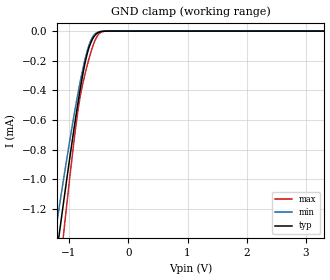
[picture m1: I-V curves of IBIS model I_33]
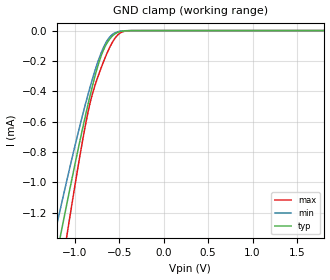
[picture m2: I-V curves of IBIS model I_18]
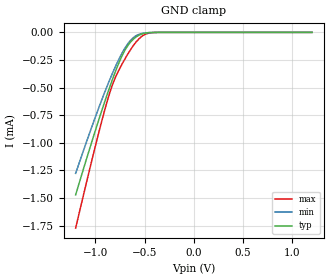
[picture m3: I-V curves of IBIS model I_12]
| TEXAS INSTRUMENTS INCORPORATED
| Standard Linear and Logic Group / High Volume Linear
| IBIS Model of TXB0304RSV, TXB0304RUT,
| 4 bit translator
| This file contains package information for the following:
|  RSV_16p 16-pin (PW) package as [Component] TXB0304RSV_PW
|  RUT_12 12-pin (PW) package as [Component] TXB0304RUT_PW
| This device can be powered at the following Vccs:
|  3.3 volt Vcc
|  1.8 volt Vcc
|  1.2 volt Vcc
| This file provides unique models under the [Model Selector] for each Vcc.
| For operation at a specific Vcc, select the appropriate model after each
| [Model Selector] keyword.
[IBIS Ver]   4.0
[Comment char]  |_char
[File Name]   txb0304.ibs
[File Rev]   1.1 | TXB0304
[Date]   June 21, 2012
[Source]   Data created from TI-SPICE simulations at TI-SLL/HVL.
   The following is an IBIS list for the TXB0304RSV and TXB0304RUT.
   Please contact sllibis@ti.com with questions and
   comments concerning SLL IBIS models.
[Notes]   Revision_History:
   - 1.1 06/21/12   Added models for one-shot circuit on for IO model
   - Non-monotonic behavior in I/O Pullup and Pulldown is expected
   -  Please note that models for one shot circuit on can be chosen under
   [Model Selector] for IO model.
[Disclaimer]
| This model is designed as an aid for customers of Texas Instruments.
| TI and its licensors and suppliers make no warranties, either expressed
| or implied, with respect to this  model, including the warranties of
| merchantability or fitness for a particular purpose. The model is
| provided solely on an "as is" basis. The entire risk as to its quality
| and performance is with the customer.
[Copyright]
| (C) Copyright 2012 Texas Instruments Incorporated. All rights reserved.
| Component TXB0304RSV_PW 16-PIN RSV_16P
[Component]   TXB0304RSV_PW
[Manufacturer]   Texas Instruments, Inc.
[Package]
|   typ   min   max
R_pkg   6.239e-02   1.070e-03   9.845e-02
L_pkg   6.891e-10   1.266e-10   1.063e-09
C_pkg   1.354e-13   8.974e-14   1.623e-13
[Pin]   signal_name   model_name   R_pin   L_pin   C_pin
1   A1   IO   7.350e-02   7.894e-10   1.363e-13
2   A2   IO   6.697e-02   7.142e-10   1.449e-13
3   A3   IO   6.675e-02   7.118e-10   1.438e-13
4   A4   IO   6.786e-02   7.288e-10   1.311e-13
5   NC   NC   1.070e-03   1.319e-10   8.974e-14
6   GND   GND   8.279e-02   8.839e-10   1.573e-13
7   GND   GND   8.757e-02   9.358e-10   1.623e-13
8   OE   I   9.845e-02   1.063e-09   1.529e-13
9   B4   IO   6.786e-02   7.222e-10   1.310e-13
10   B3   IO   6.675e-02   7.050e-10   1.436e-13
11   B2   IO   6.697e-02   7.075e-10   1.447e-13
12   B1   IO   7.350e-02   7.835e-10   1.361e-13
13   VCC   POWER   8.803e-02   9.463e-10   1.432e-13
14   NC   NC   1.070e-03   1.266e-10   1.031e-13
15   NC   NC   1.070e-03   1.266e-10   1.031e-13
16   VCC   POWER   8.803e-02   9.491e-10   1.433e-13
| Component TXB0304RUT_PW 12-PIN RUT_12
[Component]   TXB0304RUT_PW
[Manufacturer]   Texas Instruments, Inc.
[Package]
|   typ   min   max
R_pkg   6.179e-02   3.158e-02   6.816e-02
L_pkg   6.348e-10   4.117e-10   7.835e-10
C_pkg   2.231e-13   1.717e-13   2.693e-13
[Pin]   signal_name   model_name   R_pin   L_pin   C_pin
1   VCC   POWER   6.816e-02   7.779e-10   2.693e-13
2   A1   IO   6.153e-02   5.719e-10   1.863e-13
3   A2   IO   6.261e-02   5.772e-10   2.487e-13
4   A3   IO   6.455e-02   6.041e-10   1.874e-13
5   A4   IO   6.783e-02   7.745e-10   2.690e-13
6   GND   GND   3.158e-02   4.117e-10   1.880e-13
7   B4   IO   6.776e-02   7.764e-10   2.647e-13
8   B3   IO   6.455e-02   6.100e-10   1.875e-13
9   B2   IO   6.261e-02   5.835e-10   2.489e-13
10   B1   IO   6.153e-02   5.783e-10   1.865e-13
11   VCC   POWER   6.815e-02   7.835e-10   2.690e-13
12   OE   I   6.063e-02   5.684e-10   1.717e-13
| Model I
[Model Selector]   I
I_33   3.3 volt Vcc
I_18   1.8 volt Vcc
I_12   1.2 volt Vcc
| Model IO
[Model Selector]   IO
IO_33   3.3 volt Vcc
IO_18   1.8 volt Vcc
IO_12   1.2 volt Vcc
IO_33_OS   one shot circuit on at   3.3 volt Vcc
IO_18_OS   one shot circuit on at  1.8 volt Vcc
IO_12_OS   one shot circuit on at   1.2 volt Vcc
| Models and submodels in the file (9): I_33 (Input), I_18 (Input), I_12 (Input), IO_33 (3-state), IO_18 (3-state), IO_12 (3-state), IO_33_OS (I/O), IO_18_OS (I/O), IO_12_OS (I/O)
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[Model]   I_33
Model_type  Input
Vinl=1.155
Vinh=2.145
| variable   typ   min   max
C_comp   0.49pF   0.33pF   0.66pF
[Temperature Range]   40   100   -40
| Ambient temperature   25   85   -40
[Voltage range]   3.3   3   3.6
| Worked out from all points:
|   GND clamp passes 1 mA (typ) near -1.04 V on its own axis
[GND Clamp]
| I_33
|   Voltage   I(typ)   I(min)   I(max)
-3.3V     -8.236mA   -7.402mA   -10.23mA
-1.225V   -1.547mA   -1.344mA   -1.868mA
-1.16V    -1.353mA   -1.173mA   -1.622mA
-1.1V     -1.177mA   -1.018mA   -1.397mA
-1.075V   -1.104mA   -954.4uA   -1.305mA
-910mV    -642.5uA   -554.3uA   -721.3uA
-810mV    -387.9uA   -337.9uA   -438uA
-675mV    -126.6uA   -109.9uA   -203.7uA
-600mV    -51.19uA   -38.37uA   -103.3uA
-525mV    -14.23uA   -9.737uA   -34.33uA
-365mV    -261.1nA   -191.2nA   -391.1nA
3.3V      1.186nA    2.425nA    22.67pA
[Model]   I_18
Model_type  Input
Vinl=0.63
Vinh=1.17
| variable   typ   min   max
C_comp   0.53pF   0.36pF   0.72pF
[Temperature Range]   40   100   -40
| Ambient temperature   25   85   -40
[Voltage range]   1.8   1.65   1.95
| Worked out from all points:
|   GND clamp passes 1 mA (typ) near -1.04 V on its own axis
[GND Clamp]
| I_18
|   Voltage   I(typ)   I(min)   I(max)
-1.8V     -3.331mA   -2.937mA   -4.119mA
-1.22V    -1.532mA   -1.33mA    -1.85mA
-1.145V   -1.309mA   -1.134mA   -1.566mA
-1.075V   -1.104mA   -954.4uA   -1.305mA
-920mV    -669.4uA   -577.3uA   -754.3uA
-825mV    -424uA     -368.5uA   -472.8uA
-695mV    -155.3uA   -136.7uA   -234uA
-630mV    -76.03uA   -61.12uA   -140.6uA
-560mV    -27.36uA   -19.07uA   -61.57uA
-485mV    -6.022uA   -4.161uA   -14.74uA
-380mV    -401.2nA   -288.1nA   -668.7nA
1.8V      414.2pA    982.6pA    13.12pA
[Model]   I_12
Model_type  Input
Vinl=0.42
Vinh=0.78
| variable   typ   min   max
C_comp   0.55pF   0.38pF   0.76pF
[Temperature Range]   40   100   -40
| Ambient temperature   25   85   -40
[Voltage range]   1.2   1.1   1.3
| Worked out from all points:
|   GND clamp passes 1 mA (typ) near -1.04 V on its own axis
[GND Clamp]
| I_12
|   Voltage   I(typ)   I(min)   I(max)
-1.2V     -1.472mA   -1.278mA   -1.773mA
-970mV    -806.2uA   -695.1uA   -925.5uA
-895mV    -602.6uA   -520.2uA   -672.8uA
-840mV    -461.1uA   -399.8uA   -510.9uA
-780mV    -318.5uA   -279.2uA   -376.9uA
-730mV    -215.1uA   -190.4uA   -289.7uA
-685mV    -140.4uA   -122.9uA   -218.7uA
-615mV    -62.82uA   -48.77uA   -121.4uA
-535mV    -17.33uA   -11.87uA   -41.15uA
-470mV    -4.244uA   -2.944uA   -10.21uA
-380mV    -401.2nA   -288.1nA   -668.7nA
1.2V      253.6pA    676.5pA    10.32pA
